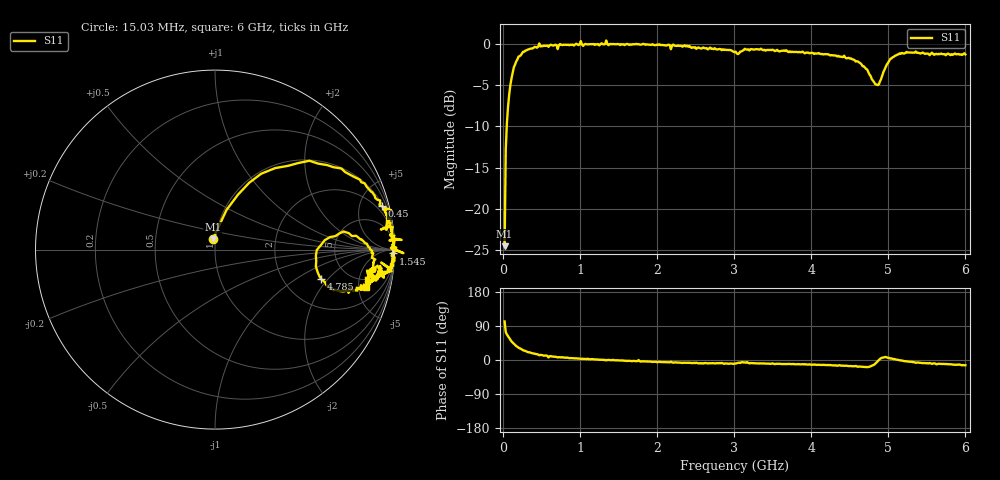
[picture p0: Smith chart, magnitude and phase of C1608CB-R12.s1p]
!	Network	Analyzer	HP8753E.07.74:	Oct	30	2002	Serial	No.	JP38451487
!	Hewlett-Packard
!	7	Sep	2009	9:55:44
!	Frequency	S11
#	HZ	S	RI	R	50
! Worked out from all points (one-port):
!   400 points, 15.03 MHz to 6 GHz, reference 50 ohm
!   lowest |S11| = -24.5 dB at 15.03 MHz (marker M1), VSWR 1.13, Z = 48.5 + j5.66 ohm
!   |S11| at or under -10 dB: start of sweep to 43.07 MHz
!   S11 on the Smith chart (normalised r, x): 15.03 MHz: 0.97, +0.11; 450 MHz: 1.22, +7.65; 1.545 GHz: 27, -85; 4.785 GHz: 3.21, -1.66; 6 GHz: 3.68, -6.02
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1.502992e7  -0.0121 0.0582
3.002985e7  0.0643 0.221
6.00297e7  0.191 0.373
9.002955e7  0.335 0.454
1.650292e8  0.624 0.471
2.550287e8  0.807 0.39
4.500278e8  0.93 0.241
5.550272e8  0.954 0.205
5.850271e8  0.954 0.11
6.150269e8  0.974 0.173
7.650262e8  0.976 0.127
1.005025e9  1.04 0.0538
1.035025e9  0.972 0.0509
1.245024e9  0.98 0.00922
1.335023e9  1.05 -0.0198
1.515022e9  0.985 -0.0204
1.545022e9  0.993 -0.0212
2.265019e9  0.973 -0.115
3.015015e9  0.886 -0.147
3.105014e9  0.906 -0.0896
3.765011e9  0.879 -0.162
4.515007e9  0.786 -0.224
4.785006e9  0.589 -0.162
4.875006e9  0.567 -0.00235
4.965005e9  0.716 0.101
5.085005e9  0.847 0.0319
5.265004e9  0.885 -0.0676
6e9  0.839 -0.207
